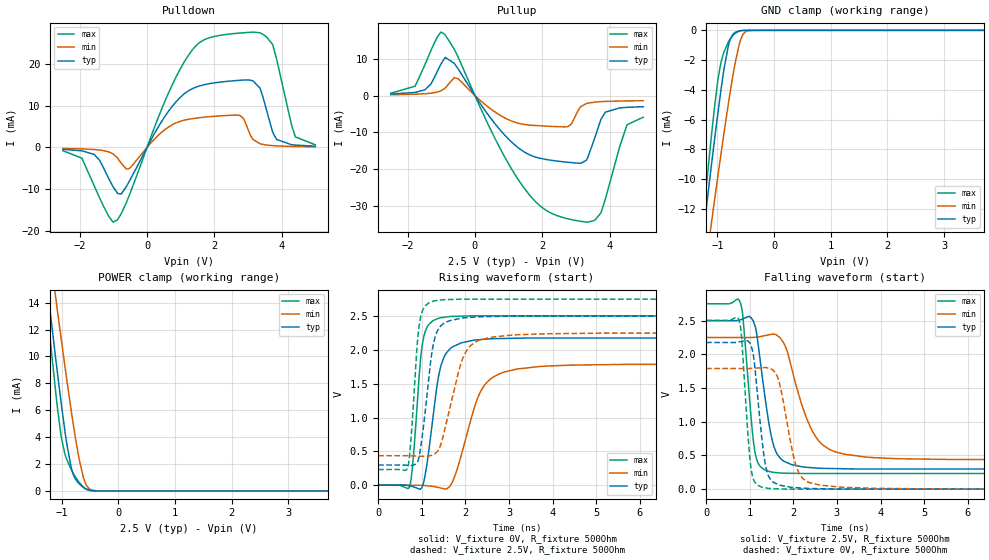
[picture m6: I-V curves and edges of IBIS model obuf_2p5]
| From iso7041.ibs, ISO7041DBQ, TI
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|   obuf_2p5 Model
[Model]   obuf_2p5
Model_type   3-state
Polarity   Non-Inverting
Vmeas = 1.25
Vref = 0
Cref = 2pF
Rref = 100000
|   typ   min   max
C_comp   0.476pF   0.446pF   0.542pF
| Where Nom  PVT is Nominal Process, 2.5V, 27C
|   Fast PVT is Strong Process,  2.75V, -55C
|   Slow PVT is Weak Process,   2.25V, 150C
[Voltage Range]   2.5   2.25   2.75
|Junction Temperature
[Temperature Range]   27   150   -55
[Pullup Reference]   2.5   2.25   2.75
[Pulldown Reference]   0   0   0
[Power Clamp Reference]   2.5   2.25   2.75
[GND Clamp Reference]   0   0   0
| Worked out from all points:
|   slope of the pulldown table from 0 to 0.375 V, typ, clamps not added: 69.1 ohm
|   slope of the pullup table from 0 to 0.375 V, typ, clamps not added: 75.2 ohm
|   GND clamp passes 1 mA (typ) near -0.81 V on its own axis
|   POWER clamp passes 1 mA (typ) near -0.77 V on its own axis
|   falling waveform, V_fixture 2.5V, R_fixture 500Ohm: 20-80 % time 301ps typ, 568ps min, 196ps max; typ from 2.5 V to 0.298 V
|   rising waveform, V_fixture 0V, R_fixture 500Ohm: 20-80 % time 284ps typ, 524ps min, 180ps max; typ from 0 V to 2.18 V
|   rising waveform, V_fixture 2.5V, R_fixture 500Ohm: 20-80 % time 246ps typ, 431ps min, 161ps max; typ from 0.298 V to 2.5 V
|   falling waveform, V_fixture 0V, R_fixture 500Ohm: 20-80 % time 213ps typ, 326ps min, 157ps max; typ from 2.18 V to 0 V
[Pulldown]
|   Voltage   I(typ)   I(min)   I(max)
-2.5V     -454uA     -235uA     -769uA
-1.938V   -807uA     -346.6uA   -2.565mA
-1.562V   -1.725mA   -507.6uA   -9.294mA
-880mV    -10.91mA   -2.479mA   -17.3mA
-557.5mV  -8.522mA   -5.154mA   -12.04mA
537.5mV   7.483mA    4.291mA    11.15mA
1.302V    13.85mA    6.815mA    22.82mA
2.757V    16.03mA    7.626mA    27.31mA
3.155V    15.85mA    1.869mA    27.54mA
3.853V    1.901mA    366.6uA    21.01mA
4.407V    553.9uA    218.6uA    2.524mA
5V        315.7uA    152.2uA    625.9uA
[GND Clamp]
|   Voltage   I(typ)   I(min)   I(max)
-2.5V     -55.83mA   -53.86mA   -64.45mA
-1.48V    -21.25mA   -23.68mA   -21.89mA
-1.218V   -12.61mA   -16.11mA   -11.33mA
-1.105V   -9.02mA    -12.92mA   -7.053mA
-1.045V   -7.159mA   -11.25mA   -4.955mA
-977.5mV  -5.141mA   -9.394mA   -2.983mA
-902.5mV  -3.066mA   -7.379mA   -1.665mA
-805mV    -991.2uA   -4.875mA   -767.6uA
-692.5mV  -148.3uA   -2.297mA   -213.3uA
-572.5mV  -14.69uA   -459.9uA   -19.13uA
-437.5mV  -623.7nA   -18.44uA   -424.3nA
5V        0A         0A         0A
[Pullup]
|   Voltage   I(typ)   I(min)   I(max)
-2.5V     398.6uA    208.5uA    640.9uA
-1.78V    848.3uA    352.8uA    2.524mA
-1.113V   6.672mA    966.6uA    15.97mA
-895mV    10.18mA    1.967mA    16.57mA
-512.5mV  7.41mA     4.618mA    10.67mA
605mV     -7.745mA   -4.516mA   -11.81mA
1.482V    -15.38mA   -7.862mA   -25.34mA
2.765V    -18.09mA   -8.412mA   -33.42mA
3.312V    -17.48mA   -2.168mA   -34.3mA
3.875V    -4.503mA   -1.589mA   -28.06mA
4.52V     -3.19mA    -1.452mA   -7.897mA
5V        -3.029mA   -1.41mA    -5.88mA
[POWER Clamp]
|   Voltage   I(typ)   I(min)   I(max)
-2.5V     62.69mA    61.31mA    69.66mA
-1.337V   18.3mA     21.98mA    17.09mA
-1.24V    14.71mA    18.78mA    12.88mA
-1.097V   9.603mA    14.16mA    7.072mA
-1V       6.29mA     11.08mA    3.86mA
-940mV    4.407mA    9.22mA     2.717mA
-827.5mV  1.68mA     5.887mA    1.568mA
-692.5mV  534.9uA    2.403mA    648.5uA
-617.5mV  267.1uA    1.024mA    296uA
-550mV    112.7uA    351uA      101.1uA
-302.5mV  343.4nA    2.682uA    50.61nA
5V        0A         0A         0A
[Ramp]
R_load = 500
|   typ   min   max
dV/dt_r   1.30546/2.8432e-10   1.07343/5.23193e-10   1.50214/1.79676e-10
dV/dt_f   1.32108/3.01279e-10   1.0887/5.68087e-10   1.5111/1.96299e-10
[Falling Waveform]
V_fixture = 2.5V
V_fixture_min = 2.25V
V_fixture_max = 2.75V
R_fixture = 500Ohm
C_fixture = 0F
|   Time   V(typ)   V(min)   V(max)
0s        2.5V       2.25V      2.75V
789.8ps   2.512V     2.249V     2.758V
1.071ns   2.507V     2.25V      795.9mV
1.202ns   2.104V     2.258V     375mV
1.5ns     771.8mV    2.297V     253.6mV
1.742ns   433.5mV    2.205V     238.2mV
2.295ns   324.5mV    1.068V     232.6mV
2.621ns   309.4mV    689.2mV    232.6mV
4.411ns   299.9mV    451.5mV    232.6mV
150ns     298.2mV    435.5mV    231.5mV
[Rising Waveform]
V_fixture = 0V
V_fixture_min = 0V
V_fixture_max = 0V
R_fixture = 500Ohm
C_fixture = 0F
|   Time   V(typ)   V(min)   V(max)
0s        -325.3nV   -338.1nV   -4.542nV
724.1ps   -9.861mV   -74.55uV   -16.57mV
974.6ps   -55.06mV   -100.2uV   1.878V
1.116ns   305.7mV    -7.725mV   2.329V
1.5ns     1.878V     -50.89mV   2.48V
1.73ns    2.052V     90.87mV    2.495V
2.165ns   2.139V     1.058V     2.502V
2.908ns   2.168V     1.676V     2.502V
5.697ns   2.174V     1.785V     2.502V
150ns     2.176V     1.789V     2.504V
[Rising Waveform]
V_fixture = 2.5V
V_fixture_min = 2.25V
V_fixture_max = 2.75V
R_fixture = 500Ohm
C_fixture = 0F
|   Time   V(typ)   V(min)   V(max)
0s        298.2mV    435.5mV    231.5mV
681.3ps   294.2mV    436.2mV    267.8mV
915.5ps   366.5mV    430mV      2.227V
1.04ns    879.9mV    426.7mV    2.613V
1.219ns   1.908V     442mV      2.707V
1.325ns   2.229V     479.9mV    2.728V
1.925ns   2.469V     1.849V     2.749V
2.621ns   2.492V     2.19V      2.749V
5.115ns   2.498V     2.246V     2.749V
150ns     2.5V       2.25V      2.75V
[Falling Waveform]
|Gnd
V_fixture = 0V
V_fixture_min = 0V
V_fixture_max = 0V
R_fixture = 500Ohm
C_fixture = 0F
|   Time   V(typ)   V(min)   V(max)
0s        2.176V     1.789V     2.504V
756.8ps   2.186V     1.789V     2.5V
809.8ps   2.192V     1.789V     2.282V
1.011ns   2.161V     1.791V     408.6mV
1.393ns   267.9mV    1.801V     15.6mV
1.647ns   72.09mV    1.648V     5.395mV
1.827ns   42.46mV    1.093V     1.111mV
2.212ns   16.03mV    160.5mV    1.11mV
3.844ns   2.168mV    12.79mV    1.106mV
150ns     -322.6nV   -339nV     -4.554nV
